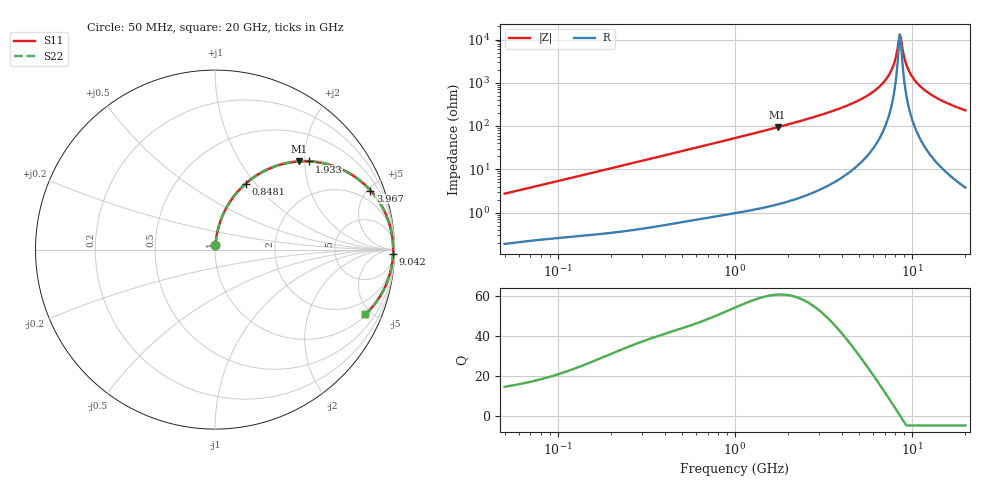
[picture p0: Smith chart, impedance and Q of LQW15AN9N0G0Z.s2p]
!Murata Part Number: LQW15AN9N0G0Z
!These Parameters are Measured in Series Mode Connection
!  o--[Z]--o
!Port1  Port2
!  o-------o
!Freq. Start=50[MHz] Stop=20[GHz], 401[Steps]
# Hz S RI R 50
!Freq.(Hz) S11(Real) S11(Imag) S21(Real) S21(Imag) S12(Real) S12(Imag) S22(Real) S22(Imag)
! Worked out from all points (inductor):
!   401 points, 50 MHz to 20 GHz, reference 50 ohm
!   read as one part in series: L = 8.6 nH near 51.52 MHz
!   highest Q = 60.9 at 1.741 GHz (marker M1), where L = 8.59 nH
!   self-resonance near 8.516 GHz
!   S11 on the Smith chart (normalised r, x): 50 MHz: 1.00, +0.05; 848.1 MHz: 1.02, +0.89; 1.933 GHz: 1.03, +2.11; 3.967 GHz: 1.12, +5.22; 9.042 GHz: 22, -72; 20 GHz: 1.08, -4.61
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5e7  0.00262 0.0271  0.9974 -0.0271  0.9974 -0.0271  0.00262 0.0271
1.364002e8  0.00806 0.0716  0.9919 -0.0716  0.9919 -0.0716  0.00806 0.0716
3.721004e8  0.0412 0.1866  0.9588 -0.1866  0.9588 -0.1866  0.0412 0.1866
8.480927e8  0.1702 0.3663  0.8298 -0.3663  0.8298 -0.3663  0.1702 0.3663
1e9  0.2211 0.4059  0.7789 -0.4059  0.7789 -0.4059  0.2211 0.4059
1.740566e9  0.4693 0.4909  0.5307 -0.4909  0.5307 -0.4909  0.4693 0.4909
1.932977e9  0.5256 0.4912  0.4744 -0.4912  0.4744 -0.4912  0.5256 0.4912
2.728004e9  0.7078 0.4459  0.2922 -0.4459  0.2922 -0.4459  0.7078 0.4459
3.967106e9  0.8662 0.3287  0.1338 -0.3287  0.1338 -0.3287  0.8662 0.3287
5.944466e9  0.9652 0.1611  0.0348 -0.1611  0.0348 -0.1611  0.9652 0.1611
6.802353e9  0.9818 0.1017  0.0182 -0.1017  0.0182 -0.1017  0.9818 0.1017
7.442007e9  0.9886 0.0618  0.0114 -0.0618  0.0114 -0.0618  0.9886 0.0618
7.901521e9  0.9913 0.0351  0.00872 -0.0351  0.00872 -0.0351  0.9913 0.0351
8.389408e9  0.9925 0.00832  0.00749 -0.00832  0.00749 -0.00832  0.9925 0.00832
8.516016e9  0.9926 0.00164  0.00741 -0.00164  0.00741 -0.00164  0.9926 0.00164
8.774992e9  0.9925 -0.0117  0.00752 0.0117  0.00752 0.0117  0.9925 -0.0117
9.041845e9  0.992 -0.0251  0.00799 0.0251  0.00799 0.0251  0.992 -0.0251
9.457416e9  0.9906 -0.0452  0.00938 0.0452  0.00938 0.0452  0.9906 -0.0452
9.892087e9  0.9884 -0.0652  0.0116 0.0652  0.0116 0.0652  0.9884 -0.0652
1.149051e10  0.975 -0.1317  0.025 0.1317  0.025 0.1317  0.975 -0.1317
1.460232e10  0.9333 -0.2359  0.0667 0.2359  0.0667 0.2359  0.9333 -0.2359
2e10  0.8378 -0.3606  0.1622 0.3606  0.1622 0.3606  0.8378 -0.3606
